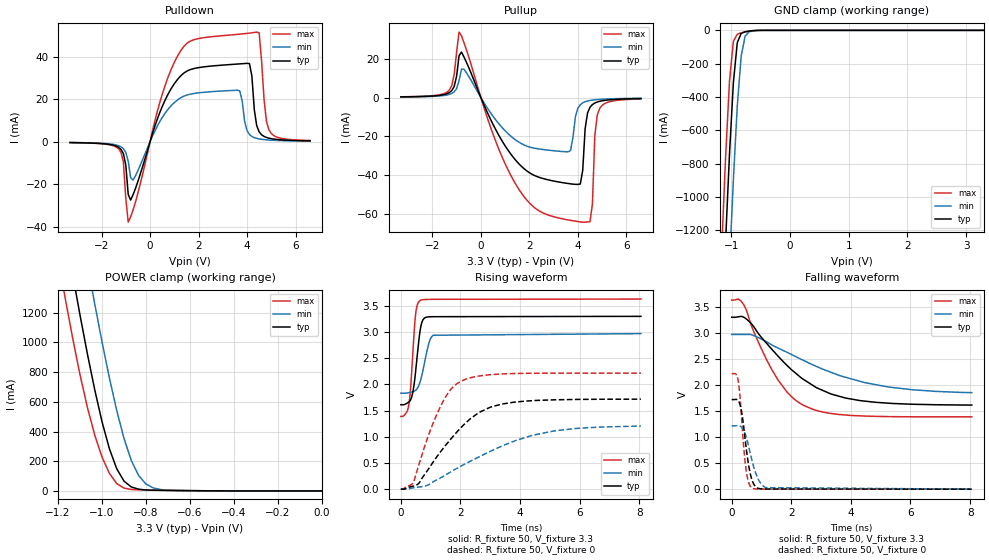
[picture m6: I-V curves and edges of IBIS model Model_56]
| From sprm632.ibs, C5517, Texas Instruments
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| Model based on original model for BC3350CTHYPU
|   Sub model PU_OFF_IND_3P3
[model]   Model_56
|[Description]  [3.3V-I/O-PU_OFF-X, IND]
|   PU_OFF,IND,
|[Input Load]   PU_OFF
|[Output Drive]
|Voltage   3.3V
|Mode   I/O
Model_type   I/O
Polarity   Non-Inverting
Enable   Active-Low
Vinl =  0.8
Vinh =  2
Cref =  15.0000pF
Rref =  100.0000M
Vref =  0V
Vmeas =  1.65
C_comp   0.87673039p  0.86952386p   1.2993811p
[Model Spec]
Vinl   0.8   0.8   0.8
Vinh   2   2   2
[Temperature Range]   25   105   -40
[Voltage Range]   3.3   2.97   3.63
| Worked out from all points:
|   slope of the pulldown table from 0 to 0.495 V, typ, clamps not added: 30.2 ohm
|   slope of the pullup table from 0 to 0.495 V, typ, clamps not added: 36.2 ohm
|   GND clamp passes 1 mA (typ) near -0.58 V on its own axis
|   POWER clamp passes 1 mA (typ) near -0.52 V on its own axis
|   rising waveform, R_fixture 50, V_fixture 3.3: 20-80 % time 199ps typ, 268ps min, 156ps max; typ from 1.61 V to 3.3 V
|   rising waveform, R_fixture 50, V_fixture 0: 20-80 % time 1.53ns typ, 2.64ns min, 921ps max; typ from 0.001 V to 1.72 V
|   falling waveform, R_fixture 50, V_fixture 3.3: 20-80 % time 1.91ns typ, 2.85ns min, 1.27ns max; typ from 3.3 V to 1.61 V
|   falling waveform, R_fixture 50, V_fixture 0: 20-80 % time 244ps typ, 350ps min, 188ps max; typ from 1.72 V to 0 V
[POWER_clamp]
-3.3V     22.37A     22.96A     21.96A
-1.2V     2.026A     2.675A     1.569A
-1.167V   1.737A     2.381A     1.292A
-1.133V   1.455A     2.091A     1.028A
-1.1V     1.183A     1.806A     781.9mA
-1.067V   923.7mA    1.529A     562.8mA
-1.033V   682.1mA    1.26A      376.9mA
-966.7mV  284.5mA    761.6mA    118.3mA
-933.3mV  149.5mA    542.1mA    49.49mA
-866.7mV  26.43mA    203.8mA    9.967mA
-800mV    6.477mA    45.96mA    6.096mA
0V        470.2pA    4.969nA    232.1pA
[Pulldown]
-3.3V     -379.4uA   -332.5uA   -396.2uA
-1.3V     -2.568mA   -1.838mA   -3.257mA
-1.1V     -5.533mA   -3.228mA   -9.383mA
-900mV    -24.8mA    -9.223mA   -37.83mA
-700mV    -24.92mA   -18.03mA   -32.09mA
500mV     16.51mA    11.37mA    22.25mA
1.3V      31.39mA    20.91mA    43.42mA
3.7V      36.65mA    23.93mA    50.64mA
4.1V      36.79mA    3.426mA    51.12mA
4.4V      7.557mA    1.597mA    51.61mA
4.9V      1.707mA    822.5uA    5.677mA
6.6V      436uA      304.4uA    587.7uA
[Pullup]
-3.3V     352.6uA    285.2uA    400.6uA
-1.3V     2.559mA    1.632mA    3.875mA
-900mV    21.62mA    8.718mA    33.78mA
1.6V      -34.58mA   -23.24mA   -47.95mA
3.7V      -44.51mA   -27.32mA   -63.35mA
4.2V      -37.49mA   -2.71mA    -64.29mA
4.3V      -15.98mA   -2.138mA   -64.26mA
4.5V      -4.997mA   -1.493mA   -64.05mA
4.6V      -3.604mA   -1.294mA   -54.92mA
4.7V      -2.803mA   -1.142mA   -19.48mA
4.9V      -1.927mA   -922.7uA   -5.592mA
6.6V      -515.4uA   -347uA     -695.9uA
[GND_clamp]
-3.3V     -22.52A    -23.16A    -22.07A
-1.167V   -1.839A    -2.548A    -1.318A
-1.1V     -1.269A    -1.966A    -766.5mA
-1.033V   -744.2mA   -1.409A    -306mA
-966.7mV  -312.6mA   -893.2mA   -65.5mA
-900mV    -73.53mA   -452.5mA   -23.28mA
-833.3mV  -18.4mA    -153.9mA   -14.52mA
-766.7mV  -8.834mA   -34.89mA   -8.497mA
-700mV    -4.682mA   -8.855mA   -4.019mA
-433.3mV  -36.27uA   -120.8uA   -8.278uA
3.3V      470.2pA    85.46uA    154.8pA
[Ramp]
dV/dt_f   1.023048/1.9214651n 0.69087744/2.9578755n   1.35676/1.270709n
dV/dt_r  1.0319626/1.5308716n 0.72982883/2.6839602n  1.3300193/0.92114554n
R_load = 50
[Rising Waveform]
R_fixture = 50
V_fixture = 3.3
V_fixture_min = 2.97
V_fixture_max = 3.63
0s        1.613V     1.833V     1.389V
249.7ps   1.658V     1.841V     1.558V
304ps     1.686V     1.849V     1.779V
361ps     1.753V     1.856V     2.219V
498ps     2.263V     1.89V      3.354V
567.1ps   2.646V     1.941V     3.542V
667.8ps   3.102V     2.094V     3.608V
923.8ps   3.289V     2.752V     3.624V
1.088ns   3.293V     2.939V     3.625V
8.057ns   3.3V       2.97V      3.63V
[Rising Waveform]
R_fixture = 50
V_fixture = 0
V_fixture_min = 0
V_fixture_max = 0
0s        596.1uV    877uV      633.4uV
417.6ps   59.03mV    26.19mV    128.6mV
901ps     364.5mV    77.7mV     988.4mV
1.35ns    728.4mV    221.3mV    1.604V
1.696ns   971.1mV    338.3mV    1.92V
2.093ns   1.22V      463.8mV    2.08V
3.004ns   1.566V     723mV      2.186V
3.776ns   1.66V      911.8mV    2.208V
5.16ns    1.707V     1.114V     2.215V
8.057ns   1.719V     1.205V     2.216V
[Falling Waveform]
R_fixture = 50
V_fixture = 3.3
V_fixture_min = 2.97
V_fixture_max = 3.63
0s        3.3V       2.971V     3.63V
369.8ps   3.31V      2.971V     3.568V
977.5ps   2.928V     2.886V     2.718V
1.554ns   2.554V     2.71V      2.097V
2.029ns   2.283V     2.579V     1.763V
2.41ns    2.107V     2.471V     1.611V
3.335ns   1.827V     2.243V     1.453V
4.318ns   1.699V     2.068V     1.407V
6.058ns   1.63V      1.909V     1.389V
8.057ns   1.614V     1.853V     1.388V
[Falling Waveform]
R_fixture = 50
V_fixture = 0
V_fixture_min = 0
V_fixture_max = 0
0s        1.72V      1.216V     2.216V
214.9ps   1.702V     1.222V     2.093V
329.3ps   1.5V       1.191V     1.384V
410.4ps   1.158V     1.12V      761.3mV
485.8ps   791.9mV    1V         361.7mV
587.2ps   399.6mV    776mV      98.25mV
711.8ps   131.2mV    484.8mV    14.57mV
932ps     9.669mV    147mV      2.669mV
1.143ns   2.803mV    29.44mV    2.034mV
8.057ns   2.771uV    47.8uV     0V
